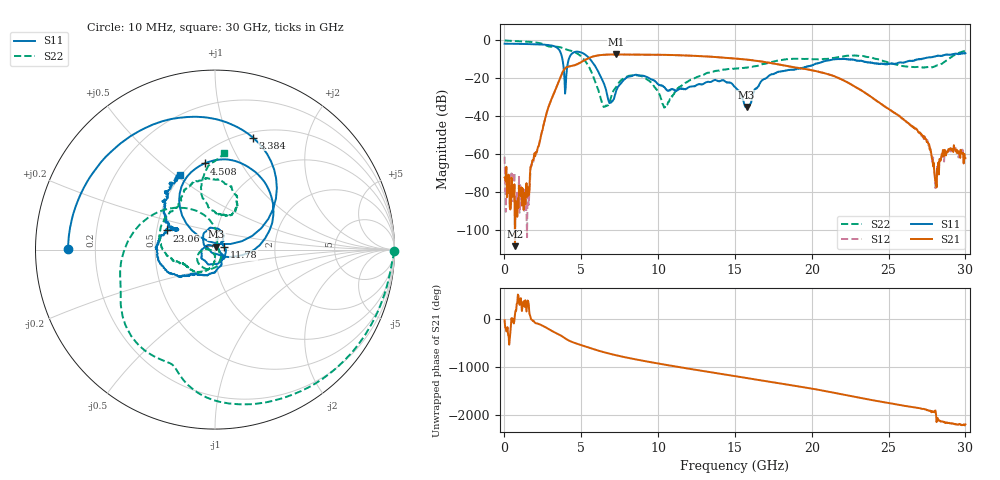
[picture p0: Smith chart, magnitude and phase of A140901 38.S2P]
!  2-Port S-parameters saved by WinCal
! VAR MeasName=S-Parameters (CALIBRATED_DATA) read from VNA (N5244A)
! VAR MeasDate=11/3/2014 9:33:34 AM
! VAR NAME=A140901 38
! VAR FILENAME=A140901 38.S2P
! VAR DATE=11/3/2014 9:33:34 AM
! VAR PHYS_PORTS=1,2
# Hz S RI R 50
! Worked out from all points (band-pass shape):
!   801 points, 10 MHz to 30 GHz, reference 50 ohm
!   highest |S21| = -7.37 dB at 7.283 GHz (marker M1); lowest = -108.3 dB at 684.8 MHz (marker M2)
!   |S21| within 3 dB of the highest: 5.227 GHz to 16.05 GHz (10.83 GHz wide, 102 % of centre)
!   lowest |S11| = -35.1 dB at 15.75 GHz (marker M3), VSWR 1.04, Z = 50.7 + j1.63 ohm
!   |S11| at or under -10 dB: 3.774 GHz to 4.184 GHz (409.5 MHz wide, 10.3 % of centre); 5.586 GHz to 21.38 GHz (15.79 GHz wide, 117 % of centre); 22.62 GHz to 26.85 GHz (4.224 GHz wide, 17.1 % of centre)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
!   |S22| runs from -35.4 to 0.0 dB; largest |S21 - S12| = 0.0031
!   S11 on the Smith chart (normalised r, x): 10 MHz: 0.10, +0.00; 3.384 GHz: 0.56, +1.23; 4.508 GHz: 0.57, +0.71; 11.78 GHz: 1.10, +0.03; 23.06 GHz: 0.57, +0.13; 30 GHz: 0.49, +0.52
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1e7  -0.8186 0.00248  0.000231 -8.87e-05  0.0007 -0.000523  0.9971 -0.00895
6.84775e8  -0.783 0.2206  -9.21e-07 3.72e-06  -1.6e-05 -2.04e-05  0.873 -0.4131
1.5095e9  -0.6521 0.465  6.67e-05 4.37e-05  0.000103 7.8e-05  0.5207 -0.7679
3.383875e9  0.2114 0.6239  0.0232 0.0535  0.023 0.0535  -0.3933 -0.5605
3.946188e9  0.0252 0.0309  0.1407 -0.1173  0.141 -0.1167  -0.5254 -0.2735
4.5085e9  -0.0585 0.48  -0.14 -0.167  -0.1391 -0.1669  -0.5034 0.00285
5.033325e9  0.2589 0.3975  -0.2723 0.0323  -0.2722 0.0316  -0.2935 0.2177
6.495338e9  0.0569 -0.0399  0.3753 0.1846  0.3754 0.1849  0.013 0.0125
7.282575e9  -0.0468 0.0134  0.3417 -0.2578  0.3413 -0.257  0.0303 -0.0524
1.001916e10  0.0449 0.0526  -0.366 0.2046  -0.3658 0.2037  -0.044 0.00177
1.046901e10  0.0363 0.0397  -0.2424 0.3386  -0.2427 0.3384  -0.0139 -0.0105
1.178108e10  0.0491 0.0154  0.2339 0.3259  0.2344 0.3266  -0.00662 -0.0762
1.5005e10  -0.0576 0.0143  -0.1332 -0.3051  -0.1328 -0.3043  -0.1525 -0.0965
1.575475e10  0.00714 0.016  -0.2784 -0.144  -0.2769 -0.1451  -0.1746 -0.0793
1.725425e10  0.00496 -0.1194  -0.159 0.2031  -0.1605 0.2014  -0.2597 -0.0406
2.002832e10  -0.1682 -0.1437  0.156 -0.0464  0.1575 -0.046  -0.2286 0.2194
2.306481e10  -0.2668 0.1066  -0.0486 0.0213  -0.0489 0.0213  -0.00548 0.3931
2.501416e10  -0.2083 0.1142  0.0117 0.0103  0.0116 0.0104  0.1197 0.2353
2.745085e10  -0.2824 0.2047  -0.000251 -0.00244  -0.000251 -0.00233  0.0363 0.1927
2.812562e10  -0.2842 0.2621  0.000135 3.75e-06  -4.76e-05 0.000172  -0.0137 0.2161
2.861296e10  -0.2727 0.3088  0.00111 -3.52e-05  0.000609 0.000216  -0.0501 0.2634
3e10  -0.1959 0.4163  0.000549 -0.000568  0.000101 -0.000746  0.0523 0.5366
